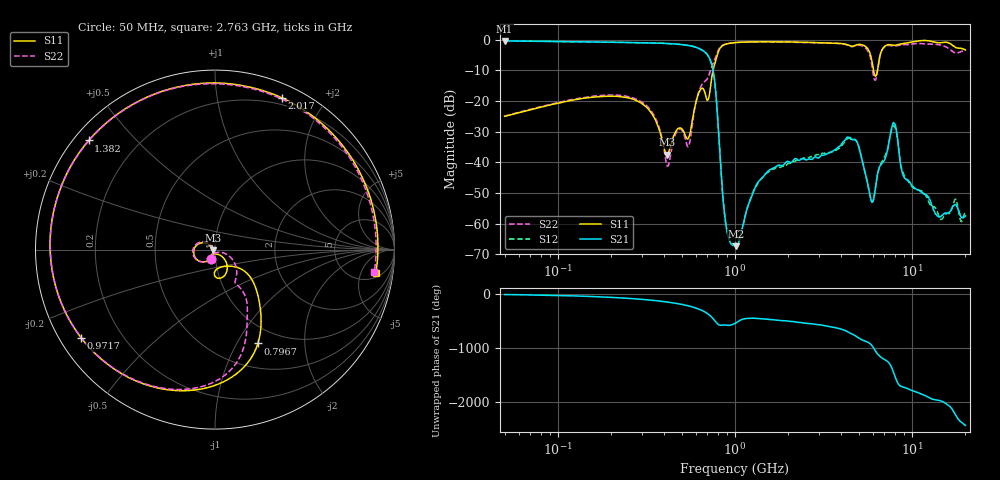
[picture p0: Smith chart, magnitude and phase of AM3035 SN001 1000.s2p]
# Hz S DB R 50
!freq MagS11 AngS11 MagS21 AngS21 MagS12 AngS12 MagS22 AngS22
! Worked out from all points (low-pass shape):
!   1601 points, 50 MHz to 20.05 GHz, reference 50 ohm
!   highest |S21| = -0.35 dB at 50 MHz (marker M1); lowest = -67.4 dB at 1.013 GHz (marker M2)
!   |S21| within 3 dB of the highest: start of sweep to 652.1 MHz
!   lowest |S11| = -37.5 dB at 413.6 MHz (marker M3), VSWR 1.03, Z = 48.7 - j0.304 ohm
!   |S11| at or under -10 dB: start of sweep to 752.6 MHz; 6.068 GHz to 6.385 GHz (317.2 MHz wide, 5.09 % of centre)
!   |S22| runs from -41.3 to -0.6 dB; largest |S21 - S12| = 0.0059
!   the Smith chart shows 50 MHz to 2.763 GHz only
!   S11 on the Smith chart (normalised r, x): 50 MHz: 0.96, -0.10; 796.7 MHz: 0.79, -1.23; 971.7 MHz: 0.06, -0.30; 1.382 GHz: 0.04, +0.37; 2.017 GHz: 0.13, +1.53; 2.763 GHz: 6, -9
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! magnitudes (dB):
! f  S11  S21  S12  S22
! 50 MHz  -25.0  -0.3  -0.4  -24.8
! 135.9 MHz  -19.2  -0.6  -0.6  -18.9
! 369.6 MHz  -28.5  -1.1  -1.1  -27.9
! 413.6 MHz  -37.5  -1.2  -1.2  -41.0
! 547.8 MHz  -32.0  -1.8  -1.8  -34.7
! 701.4 MHz  -19.7  -4.9  -5.0  -12.5
! 796.7 MHz  -4.8  -24.4  -24.3  -4.1
! 878.2 MHz  -1.5  -58.0  -57.9  -1.4
! 971.7 MHz  -1.0  -67.1  -66.7  -1.0
! 1.005 GHz  -0.9  -67.3  -66.6  -0.9
! 1.013 GHz  -0.9  -67.4  -66.4  -0.9
! 1.382 GHz  -0.6  -45.9  -46.0  -0.6
! 2.017 GHz  -0.7  -39.8  -40.4  -0.7
! 2.722 GHz  -0.8  -39.1  -38.2  -0.9
! 2.763 GHz  -0.9  -38.8  -37.9  -1.0
! 4.775 GHz  -1.8  -32.6  -32.6  -1.9
! 5.956 GHz  -7.1  -53.0  -53.0  -8.7
! 7.402 GHz  -1.6  -33.8  -33.9  -1.8
! 7.978 GHz  -1.8  -27.5  -28.3  -2.0
! 9.061 GHz  -1.2  -45.1  -44.4  -1.6
! 14.53 GHz  -0.9  -57.8  -58.6  -1.7
! 20.05 GHz  -3.3  -57.5  -56.1  -3.6
